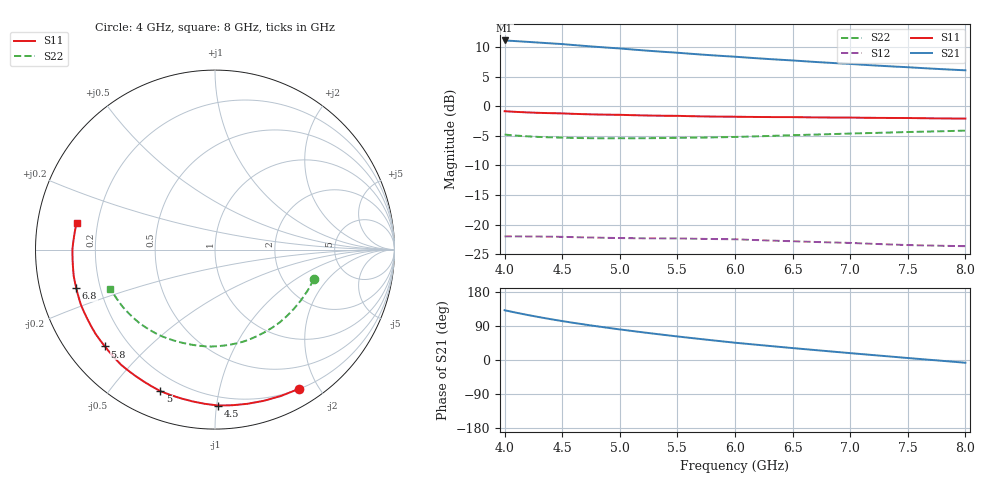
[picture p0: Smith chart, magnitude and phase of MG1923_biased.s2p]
! AWR Design Environment (7015) Thu Jan 15 11:32:17 2015
! Simulator: Linear circuit simulator
! Ports: 2, Freqs: 41
# GHz S MA R 50
!Freq  MagS11  AngS11  MagS21  AngS21  MagS12  AngS12  MagS22  AngS22
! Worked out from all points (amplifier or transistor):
!   41 points, 4 GHz to 8 GHz, reference 50 ohm
!   highest |S21| = 11.1 dB at 4 GHz (marker M1)
!   |S21| within 3 dB of that: start of sweep to 6.188 GHz
!   unconditionally stable (mu >= 1): nowhere
!   at 4.6 GHz: K = 0.45, MSG = 16.2 dB, |S12| = -22.1 dB
!   at 6 GHz: K = 0.59, MSG = 15.4 dB, |S12| = -22.5 dB
!   at 8 GHz: K = 0.81, MSG = 14.8 dB, |S12| = -23.6 dB
!   lowest NFmin = 0.85 dB at 4 GHz
!   S11 on the Smith chart (normalised r, x): 4 GHz: 0.20, -1.75; 4.5 GHz: 0.14, -1.01; 5 GHz: 0.12, -0.68; 5.8 GHz: 0.11, -0.37; 6.8 GHz: 0.11, -0.13; 8 GHz: 0.12, +0.10
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4  0.9059 -58.9  3.582 131.3  0.07969 59.5  0.5755 -16.7
4.1  0.8945 -65.8  3.535 124.8  0.07969 53.5  0.5644 -23.9
4.2  0.8852 -72.1  3.486 118.8  0.07957 48.0  0.556 -30.6
4.3  0.878 -78.1  3.435 113.1  0.0794 42.9  0.5497 -36.9
4.4  0.8725 -83.6  3.386 107.8  0.07919 38.1  0.5454 -42.8
4.5  0.8688 -88.9  3.338 102.7  0.07897 33.6  0.5427 -48.5
4.7  0.855 -98.4  3.218 93.4  0.07812 25.3  0.5372 -58.7
4.8  0.8504 -102.8  3.164 89.0  0.07774 21.5  0.536 -63.5
5  0.8451 -111.1  3.067 80.7  0.07712 14.3  0.5364 -72.5
5.2  0.8351 -118.6  2.957 73.0  0.07677 7.6  0.5362 -80.8
5.4  0.8295 -125.7  2.864 65.7  0.07662 1.4  0.5385 -88.5
5.6  0.8236 -132.4  2.773 58.7  0.07624 -4.5  0.5415 -95.7
5.8  0.8171 -138.7  2.686 52.1  0.07569 -10.1  0.5448 -102.5
6  0.8144 -144.8  2.612 45.6  0.07533 -15.4  0.5497 -108.9
6.2  0.8101 -150.0  2.531 39.9  0.07408 -20.0  0.5567 -114.8
6.4  0.8082 -155.0  2.461 34.3  0.07299 -24.4  0.5646 -120.5
6.7  0.8036 -162.3  2.359 26.1  0.07147 -30.8  0.5757 -128.5
6.8  0.8022 -164.6  2.327 23.4  0.071 -32.8  0.5795 -131.1
7  0.8008 -169.3  2.27 18.1  0.07017 -36.9  0.5876 -136.2
7.4  0.7945 -178.2  2.154 7.8  0.06782 -44.7  0.6011 -145.9
7.6  0.7915 177.5  2.102 2.8  0.06696 -48.6  0.6079 -150.6
8  0.7854 168.9  2.006 -7.2  0.06587 -56.1  0.6216 -159.6
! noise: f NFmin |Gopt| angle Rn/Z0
4  0.8482  0.6224  -1.056  0.4077
4.4  0.8745  0.5934  22.34  0.3805
4.8  0.914  0.5753  41.96  0.3524
5.3  0.972  0.5634  62.76  0.3162
5.7  1.022  0.5603  77.19  0.2868
6.2  1.086  0.5623  93.14  0.25
6.6  1.139  0.5674  104.6  0.2209
7.1  1.205  0.577  117.5  0.1855
7.5  1.258  0.5869  127  0.1585
8  1.324  0.6015  137.9  0.1268
